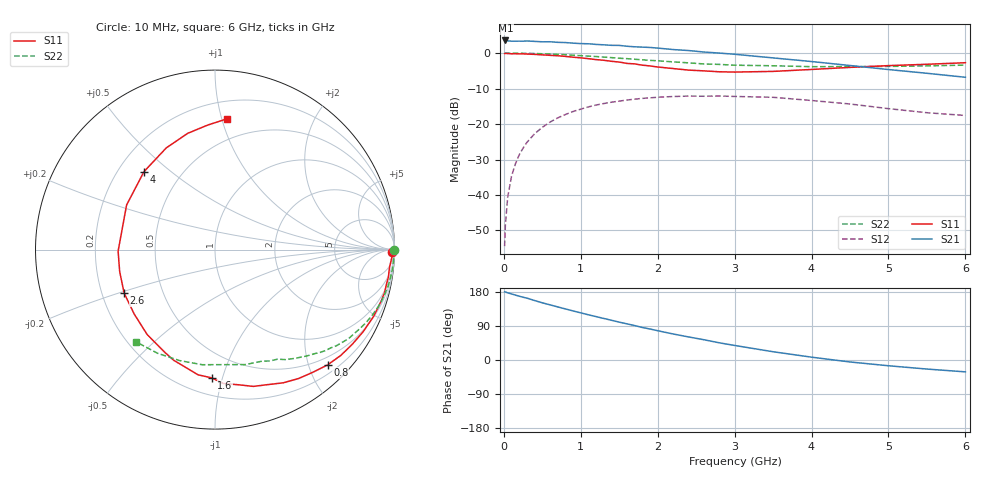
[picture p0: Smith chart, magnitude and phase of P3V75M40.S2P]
! SIEMENS Small Signal Semiconductors
! BFP181
! Si NPN RF Bipolar Junction Transistor in SOT143
! VCE = 0.75 V  IC = 0.4 mA
! Common Emitter S-Parameters:  March  1996
# GHz  S  MA  R  50
!  f  S11  S21  S12  S22
! GHz  MAG  ANG  MAG  ANG  MAG  ANG  MAG  ANG
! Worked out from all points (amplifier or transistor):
!   36 points, 10 MHz to 6 GHz, reference 50 ohm
!   highest |S21| = 3.6 dB at 20 MHz (marker M1)
!   |S21| within 3 dB of that: start of sweep to 2.477 GHz
!   unconditionally stable (mu >= 1): 3.658 GHz to end of sweep
!   at 250 MHz: K = 0.09, MSG = 15.1 dB, |S12| = -26.8 dB
!   at 1.4 GHz: K = 0.48, MSG = 8.0 dB, |S12| = -13.8 dB
!   at 6 GHz: K = 1.65, MAG = 0.7 dB, |S12| = -17.6 dB
!   S11 on the Smith chart (normalised r, x): 10 MHz: open; 800 MHz: 0.35, -2.33; 1.6 GHz: 0.32, -0.92; 2.6 GHz: 0.29, -0.21; 4 GHz: 0.31, +0.41; 6 GHz: 0.33, +1.04
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0.01  0.9841 -0.7  1.49 179.8  0.0019 87.0  0.9982 -0.2
0.02  0.9912 -1.2  1.506 179.6  0.0038 84.4  0.9974 -0.6
0.05  0.9857 -2.7  1.488 177.2  0.0093 88.9  0.9979 -1.5
0.1  0.9773 -5.8  1.469 174.4  0.0184 84.7  0.9967 -3.0
0.15  0.9782 -8.9  1.471 171.3  0.0274 83.3  0.9957 -4.5
0.2  0.9746 -11.5  1.474 168.4  0.0369 81.8  0.9954 -6.0
0.3  0.9689 -17.3  1.482 163.3  0.0552 77.3  0.9902 -9.0
0.4  0.959 -22.8  1.461 156.9  0.0729 73.4  0.986 -11.9
0.6  0.9296 -34.4  1.444 145.6  0.1065 64.6  0.9694 -17.8
0.8  0.8977 -45.7  1.407 134.8  0.1361 56.5  0.9464 -23.3
1.1  0.8339 -62.9  1.352 119.2  0.1744 45.0  0.9065 -31.0
1.5  0.7476 -86.5  1.283 99.9  0.2102 31.1  0.8457 -40.4
1.6  0.715 -91.4  1.248 95.4  0.218 28.3  0.8347 -42.3
1.9  0.6584 -110.4  1.2 81.8  0.2339 19.0  0.7889 -48.3
2.2  0.6054 -128.7  1.121 68.7  0.2441 10.9  0.7518 -53.7
2.6  0.5614 -154.4  1.035 53.5  0.2463 1.3  0.7027 -60.3
3  0.5399 -179.1  0.962 38.4  0.2447 -8.4  0.6747 -67.1
3.5  0.5517 153.2  0.855 21.8  0.2381 -17.8  0.6624 -75.3
4  0.5876 132.3  0.76 7.5  0.2146 -25.9  0.6431 -85.4
4.5  0.6283 115.6  0.668 -5.2  0.1916 -32.8  0.6453 -96.3
5.5  0.6952 93.3  0.519 -23.9  0.1444 -34.5  0.6604 -119.0
6  0.7314 84.8  0.456 -31.3  0.132 -30.8  0.6764 -130.6
